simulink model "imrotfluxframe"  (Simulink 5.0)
settings: Solver=ode45  StartTime=0.0  StopTime=1  MaxStep=2e-4  RelTol=1e-3  AbsTol=1e-3
InitFcn:
  | imdefrotflux
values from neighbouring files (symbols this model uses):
  an = atan2(phiqr,phidr)    [imdefrotflux.m]
  Bm = 0.10    (= 0.1)    [IMabc2.m]    (also in imabcparam.m = 0.01; IMabcrun0.m = 0.01; IMabcrun1.m = 0.001; IMcur0.m = 1e-06)
  fr0 = [phidr phiqr]    [imdef0vec.m]    (also in imdef1vec.m; imdefrotflux.m = sqrt(phidr^2+phiqr^2); imdefSIvec1.m)
  fs0 = fs    [calc0.m]    (also in imdef0vec.m = [phids phiqs]; imdef1vec.m = [phids phiqs]; imdefrotflux.m = [fs0d fs0q]; imdefSIvec1.m = [phids phiqs])
  H = 0.60    (= 0.6)    [IMabc2.m]    (also in IMcur0.m = 0.3; imdef0vec.m = 0.3; imdef1vec.m = 0.3; imdef2vec.m = 0.3)
  Lm = eval(get(hLm,'String'))    [im3d.m]    (also in IMabc2.m = 4.5; imabcparam.m = 0.0847; IMabcrun0.m = 0.0847; IMabcrun1.m = 0.0847)
  Lrl = eval(get(hLr,'String'))    [im3d.m]    (also in IMabc2.m = 0.1; imabcparam.m = 0.0025; IMabcrun0.m = 0.0025; IMabcrun1.m = 0.0025)
  Lsl = eval(get(hLs,'String'))    [im3d.m]    (also in IMabc2.m = 0.1; imabcparam.m = 0.0025; IMabcrun0.m = 0.0025; IMabcrun1.m = 0.0025)
  n0 = 0.98    [imdef0vec.m]    (also in imdef1vec.m = 0.978; imdef2vec.m; imdefrotflux.m; imdefSIvec1.m = 0.95)
  Rr = input('Rotor resistance)[default = 2] =')    [Actac.m]    (also in im1phase.m = 0.3; im3d.m = eval(get(hRr,'String')); IMabc2.m = 0.02; imabcparam.m = 0.408)
  Rs = eval(get(hRs,'String'))    [im3d.m]    (also in IMabc2.m = 0.01; imabcparam.m = 0.531; IMabcrun0.m = 0.531; IMabcrun1.m = 0.531)
  Tl0 = Is*conj(Is)*Req    [imdef0vec.m]    (also in imdef1vec.m; imdef2vec.m = Lm*(I(2)*I(3)-I(1)*I(4)); imdefrotflux.m; imdefSIvec1.m = Te0/To)
  vs = 1.0    (= 1)    [imdef0vec.m]    (also in imdef1vec.m; imdef2vec.m; imdefrotflux.m; imdefSIvec1.m)
  wo = 2*pi*freq0    [calc0.m]    (also in IMabc2.m = 376.991118431; imabcparam.m = 376.991118431; IMabcrun0.m = 376.991118431; IMabcrun1.m = 376.991118431)
  ws = 1.0    (= 1)    [IMabc2.m]    (also in IMcur0.m; imdef0vec.m; imdef1vec.m; imdef2vec.m)

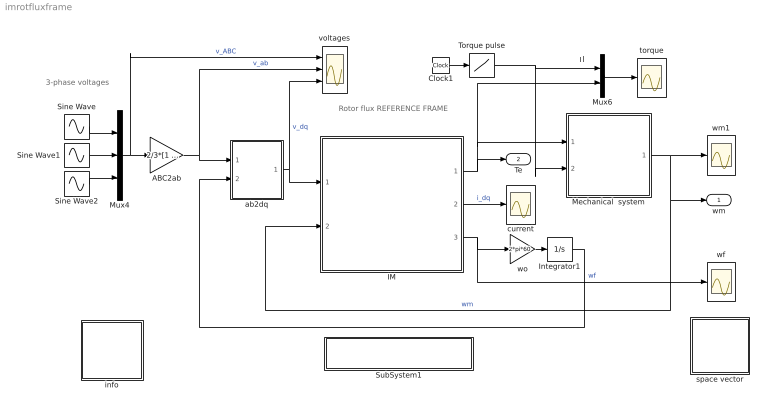
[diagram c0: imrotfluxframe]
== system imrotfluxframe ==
  note: Rotor flux REFERENCE FRAME
  note: Tl
  note: 3-phase voltages
  ABC2ab : Gain  Gain=2/3*[1 -0.5 -0.5;0 sqrt(3)/2 -sqrt(3)/2]  Multiplication=Matrix(K*u)
  Clock1 : Clock
  IM : Subsystem
  Integrator1 : Integrator
  Mechanical  system : Subsystem
  Mux4 : Mux  Inputs=3
  Mux6 : Mux  Inputs=2
  Sine Wave : Sin  Amplitude=vs  Frequency=wo*ws  Phase=pi/2-an  SampleTime=0
  Sine Wave1 : Sin  Amplitude=vs  Frequency=wo*ws  Phase=pi/2-an-2*pi/3  SampleTime=0
  Sine Wave2 : Sin  Amplitude=vs  Frequency=wo*ws  Phase=pi/2-an+2*pi/3  SampleTime=0
  SubSystem1 : Subsystem
  Torque pulse : Lookup  InputValues=[0 0.1 0.1 0.5 0.5 2]  OutputValues="[Tl0 Tl0  0 0 0.5 0.5]"
  ab2dq : Subsystem
  current : Scope
  info : Subsystem
  space vector : Subsystem
  torque : Scope
  voltages : Scope  NumInputPorts=3
  wf : Scope
  wm1 : Scope
  wo : Gain  Gain=2*pi*60
  wm : Outport
  Te : Outport  Port=2
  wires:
  Mux6/1 -> torque/1
  Torque pulse/1 -> Mux6/1, Mechanical  system/2(Tl)  "Tl"
  Mechanical  system/1(wm) -> wm1/1, IM/2(wm), wm/1  "wm"
  ab2dq/1(dq) -> IM/1(vs), voltages/3  "v_dq"
  Mux4/1 -> ABC2ab/1, voltages/1  "v_ABC"
  ABC2ab/1 -> ab2dq/1(ab), voltages/2  "v_ab"
  IM/2(is) -> current/1  "i_dq"
  IM/1(Te) -> Te/1, Mux6/2, Mechanical  system/1(Te)
  Sine Wave/1 -> Mux4/1
  Sine Wave1/1 -> Mux4/2
  Sine Wave2/1 -> Mux4/3
  Clock1/1 -> Torque pulse/1
  wo/1 -> Integrator1/1
  IM/3(wf) -> wo/1, wf/1  "wf"
  Integrator1/1 -> ab2dq/2(thetak)

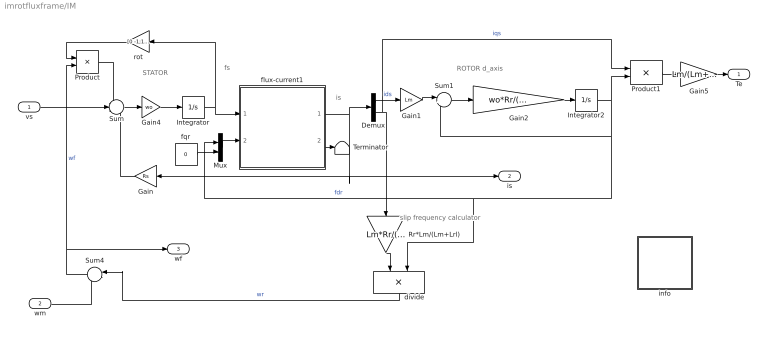
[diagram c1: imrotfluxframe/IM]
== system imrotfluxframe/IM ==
  note: STATOR
  note: fs
  note: is
  note: ROTOR d_axis
  note: slip frequency calculator
  vs : Inport
  wm : Inport  Port=2
  Demux : Demux  Outputs=2
  Gain : Gain  Orientation=left  Gain=Rs
  Gain1 : Gain  Gain=Lm
  Gain2 : Gain  Gain=wo*Rr/(Lm+Lrl)
  Gain4 : Gain  Gain=wo
  Gain5 : Gain  Gain=Lm/(Lm+Lrl)
  Integrator : Integrator  InitialCondition=fs0
  Integrator2 : Integrator  InitialCondition=fr0
  Mux : Mux  Inputs=2
  Product : Product
  Product1 : Product
  Rr*Lm/(Lm+Lrl) : Gain  Orientation=down  Gain=Lm*Rr/(Lm+Lrl)
  Sum : Sum  Inputs=-+-
  Sum1 : Sum  Inputs=|+-
  Sum4 : Sum  Orientation=left  Inputs=|++
  Terminator : Terminator
  divide : Product  Orientation=down  Inputs=*/
  flux-current1 : Subsystem
  fqr : Constant  Value=0
  info : Subsystem
  rot : Gain  Orientation=left  Gain=[0 -1;1 0]  Multiplication=Matrix(K*u)
  Te : Outport
  is : Outport  Port=2
  wf : Outport  Port=3
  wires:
  Gain/1 -> Sum/3
  Integrator/1 -> flux-current1/1(fs), rot/1
  Product/1 -> Sum/1
  rot/1 -> Product/1
  Sum/1 -> Gain4/1
  Gain4/1 -> Integrator/1
  flux-current1/1(is) -> Gain/1, is/1, Demux/1
  vs/1 -> Sum/2
  wm/1 -> Sum4/2
  Rr*Lm/(Lm+Lrl)/1 -> divide/1
  Demux/1 -> Gain1/1  "ids"
  Sum4/1 -> wf/1, Product/2  "wf"
  divide/1 -> Sum4/1  "wr"
  Mux/1 -> flux-current1/2(fr)
  fqr/1 -> Mux/2
  Demux/2 -> Rr*Lm/(Lm+Lrl)/1, Product1/1  "iqs"
  Gain1/1 -> Sum1/1
  Sum1/1 -> Gain2/1
  Gain2/1 -> Integrator2/1
  Integrator2/1 -> divide/2, Mux/1, Sum1/2, Product1/2  "fdr"
  Product1/1 -> Gain5/1
  Gain5/1 -> Te/1
  flux-current1/2(ir) -> Terminator/1

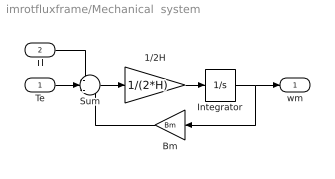
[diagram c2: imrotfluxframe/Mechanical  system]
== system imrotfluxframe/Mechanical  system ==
  Te : Inport
  Tl : Inport  Port=2
  1/2H : Gain  Gain=1/(2*H)
  Bm : Gain  Orientation=left  Gain=Bm
  Integrator : Integrator  InitialCondition=n0
  Sum : Sum  Inputs=-+-
  wm : Outport
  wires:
  1/2H/1 -> Integrator/1
  Sum/1 -> 1/2H/1
  Bm/1 -> Sum/3
  Integrator/1 -> Bm/1, wm/1
  Te/1 -> Sum/2
  Tl/1 -> Sum/1

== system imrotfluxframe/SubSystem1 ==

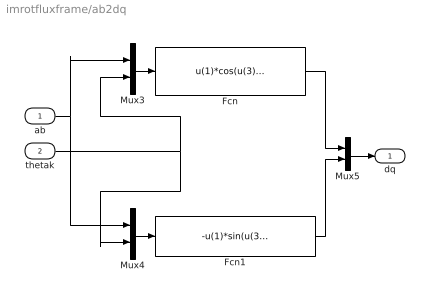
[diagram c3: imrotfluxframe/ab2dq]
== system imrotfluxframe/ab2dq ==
  ab : Inport
  thetak : Inport  Port=2
  Fcn : Fcn  Expr=u(1)*cos(u(3))+u(2)*sin(u(3))
  Fcn1 : Fcn  Expr=-u(1)*sin(u(3))+u(2)*cos(u(3))
  Mux3 : Mux  Inputs=2
  Mux4 : Mux  Inputs=2
  Mux5 : Mux  Inputs=2
  dq : Outport
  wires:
  Mux3/1 -> Fcn/1
  Mux4/1 -> Fcn1/1
  ab/1 -> Mux3/1, Mux4/1
  thetak/1 -> Mux3/2, Mux4/2
  Fcn1/1 -> Mux5/2
  Fcn/1 -> Mux5/1
  Mux5/1 -> dq/1

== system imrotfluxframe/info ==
  note: Running of an Induction Motor Modeled in the Rotor Flux Frame under Three-Phase Sinusoidal Excitation

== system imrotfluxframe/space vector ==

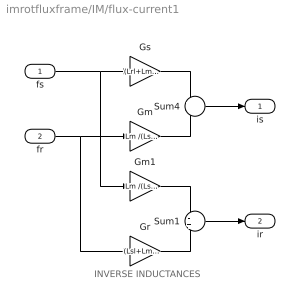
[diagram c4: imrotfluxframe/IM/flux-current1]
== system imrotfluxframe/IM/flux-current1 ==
  note: INVERSE INDUCTANCES
  fs : Inport
  fr : Inport  Port=2
  Gm : Gain  Gain=Lm /(Lsl*Lrl+Lsl*Lm+Lrl*Lm)
  Gm1 : Gain  Gain=Lm /(Lsl*Lrl+Lsl*Lm+Lrl*Lm)
  Gr : Gain  Gain=(Lsl+Lm )/(Lsl*Lrl+Lsl*Lm+Lrl*Lm)
  Gs : Gain  Gain=(Lrl+Lm) /(Lsl*Lrl+Lsl*Lm+Lrl*Lm)
  Sum1 : Sum  Inputs=-+
  Sum4 : Sum  Inputs=+-
  is : Outport
  ir : Outport  Port=2
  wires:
  fs/1 -> Gs/1, Gm1/1
  Gs/1 -> Sum4/1
  fr/1 -> Gm/1, Gr/1
  Gm/1 -> Sum4/2
  Sum4/1 -> is/1
  Gm1/1 -> Sum1/1
  Gr/1 -> Sum1/2
  Sum1/1 -> ir/1

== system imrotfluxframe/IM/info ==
  note: Mathematical model of the induction machine described in the rotor flux reference frame. (Per unit formulation)
  note: Electrical system equations: vs = Rs.is + 1/wo.(dfs/dt) + wkM(pi/2).fs where the variables is, vs, and fs are 2-dimensional space vectors and M=[0 -1;1 0] represents a 90o space rotator wf = wm + wr; wr = Rr. Lm/(Lm+Lrl). (iqs / fdr) 1/wo.(Lm+Lrl)/Rr.(dfdr/dt) +fdr = Lm.ids fqr = 0 The flux linkage current relations : fs = Ls.is + Lm.ir is = Gs.fs - Gm.fr fr = Lm.is + Lr.ir ir = Gr.fr - Gm.is Mechanical system equations: Te = 2H.dwm/dt + Bm.wm + Tl where Te = (iqs.fdr). Lm/(Lm + Lrl)
